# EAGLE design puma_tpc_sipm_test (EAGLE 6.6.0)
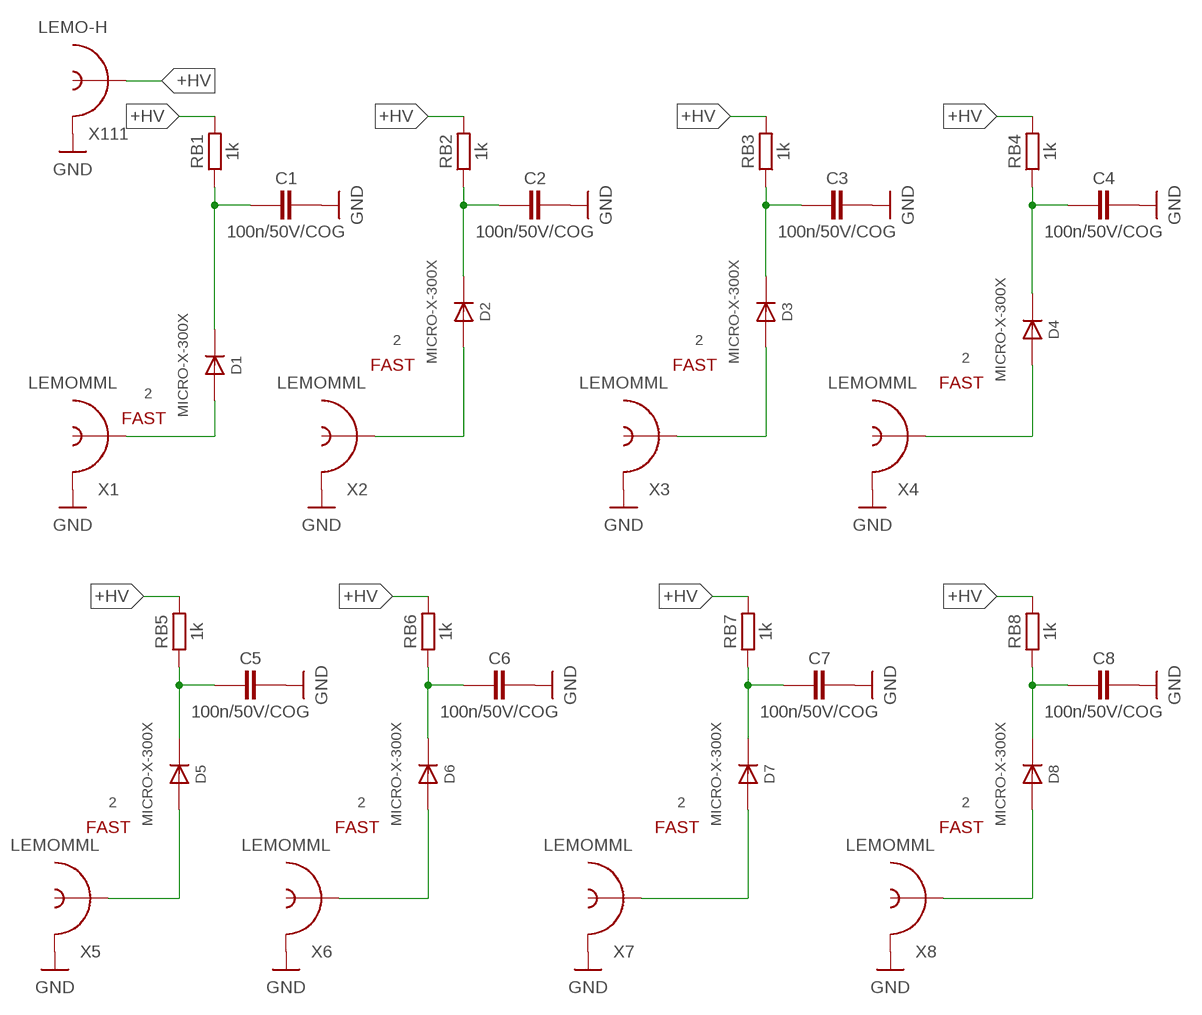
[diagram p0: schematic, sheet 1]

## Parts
C1  100n/50V/COG  C-EUCAP3216X130N  [CAP3216X130N]
C2  100n/50V/COG  C-EUCAP3216X130N  [CAP3216X130N]
C3  100n/50V/COG  C-EUCAP3216X130N  [CAP3216X130N]
C4  100n/50V/COG  C-EUCAP3216X130N  [CAP3216X130N]
C5  100n/50V/COG  C-EUCAP3216X130N  [CAP3216X130N]
C6  100n/50V/COG  C-EUCAP3216X130N  [CAP3216X130N]
C7  100n/50V/COG  C-EUCAP3216X130N  [CAP3216X130N]
C8  100n/50V/COG  C-EUCAP3216X130N  [CAP3216X130N]
D1  MICRO-X-300X  [MICROX-300XX]
D2  MICRO-X-300X  [MICROX-300XX]
D3  MICRO-X-300X  [MICROX-300XX]
D4  MICRO-X-300X  [MICROX-300XX]
D5  MICRO-X-300X  [MICROX-300XX]
D6  MICRO-X-300X  [MICROX-300XX]
D7  MICRO-X-300X  [MICROX-300XX]
D8  MICRO-X-300X  [MICROX-300XX]
RB1  1k  R-EU_RES1608X55N  [RES1608X55N]
RB2  1k  R-EU_RES1608X55N  [RES1608X55N]
RB3  1k  R-EU_RES1608X55N  [RES1608X55N]
RB4  1k  R-EU_RES1608X55N  [RES1608X55N]
RB5  1k  R-EU_RES1608X55N  [RES1608X55N]
RB6  1k  R-EU_RES1608X55N  [RES1608X55N]
RB7  1k  R-EU_RES1608X55N  [RES1608X55N]
RB8  1k  R-EU_RES1608X55N  [RES1608X55N]
X1  LEMOMML  [R302.302.000]
X2  LEMOMML  [R302.302.000]
X3  LEMOMML  [R302.302.000]
X4  LEMOMML  [R302.302.000]
X5  LEMOMML  [R302.302.000]
X6  LEMOMML  [R302.302.000]
X7  LEMOMML  [R302.302.000]
X8  LEMOMML  [R302.302.000]
X111  LEMO-H  [LEMO-H]

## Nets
+HV: RB1.2 RB2.2 RB3.2 RB4.2 RB5.2 RB6.2 RB7.2 RB8.2 X111.INNER
A1: D1.1(A) X1.1(INNER)
A2: D2.1(A) X2.1(INNER)
A3: D3.1(A) X3.1(INNER)
A4: D4.1(A) X4.1(INNER)
A5: D5.1(A) X5.1(INNER)
A6: D6.1(A) X6.1(INNER)
A7: D8.1(A) X8.1(INNER)
A8: D7.1(A) X7.1(INNER)
FILT1: C1.1 D1.3(K) RB1.1
FILT2: C2.1 D2.3(K) RB2.1
FILT3: C5.1 D5.3(K) RB5.1
FILT4: C6.1 D6.3(K) RB6.1
FILT9: C3.1 D3.3(K) RB3.1
FILT10: C4.1 D4.3(K) RB4.1
FILT11: C8.1 D8.3(K) RB8.1
FILT12: C7.1 D7.3(K) RB7.1
GND: C1.2 C2.2 C3.2 C4.2 C5.2 C6.2 C7.2 C8.2 X1.GND@1(SHIELD) X1.GND@2(SHIELD) X1.GND@3(SHIELD) X2.GND@1(SHIELD) X2.GND@2(SHIELD) X2.GND@3(SHIELD) X3.GND@1(SHIELD) X3.GND@2(SHIELD) X3.GND@3(SHIELD) X4.GND@1(SHIELD) X4.GND@2(SHIELD) X4.GND@3(SHIELD) X5.GND@1(SHIELD) X5.GND@2(SHIELD) X5.GND@3(SHIELD) X6.GND@1(SHIELD) X6.GND@2(SHIELD) X6.GND@3(SHIELD) X7.GND@1(SHIELD) X7.GND@2(SHIELD) X7.GND@3(SHIELD) X8.GND@1(SHIELD) X8.GND@2(SHIELD) X8.GND@3(SHIELD) X111.SHIELD@1(SHIELD) X111.SHIELD@2(SHIELD) X111.SHIELD@3(SHIELD) X111.SHIELD@4(SHIELD)
Unconnected: D1.2(FAST) D1.4(NC) D2.2(FAST) D2.4(NC) D3.2(FAST) D3.4(NC) D4.2(FAST) D4.4(NC) D5.2(FAST) D5.4(NC) D6.2(FAST) D6.4(NC) D7.2(FAST) D7.4(NC) D8.2(FAST) D8.4(NC)

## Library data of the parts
C1-C8 = rcl:C-EU: CAPACITOR, European symbol
D1-D8 = local:MICRO*-?: MPPC Diode with Fast output
RB1-RB8 = rcl:R-EU_: RESISTOR, European symbol
X1-X8 X111 = local:LEMO

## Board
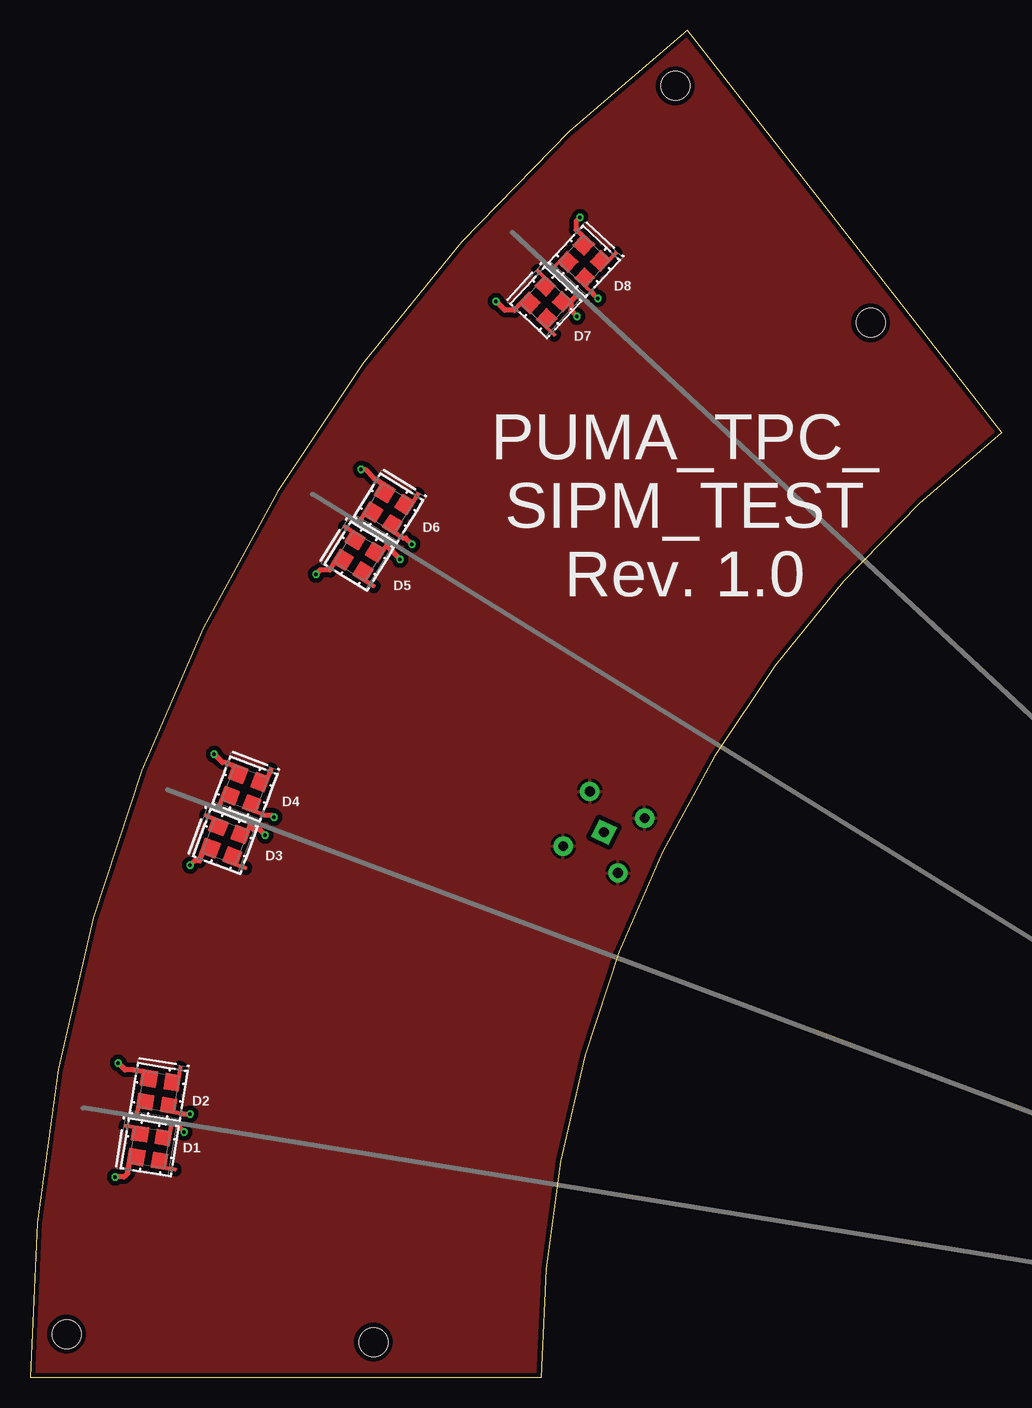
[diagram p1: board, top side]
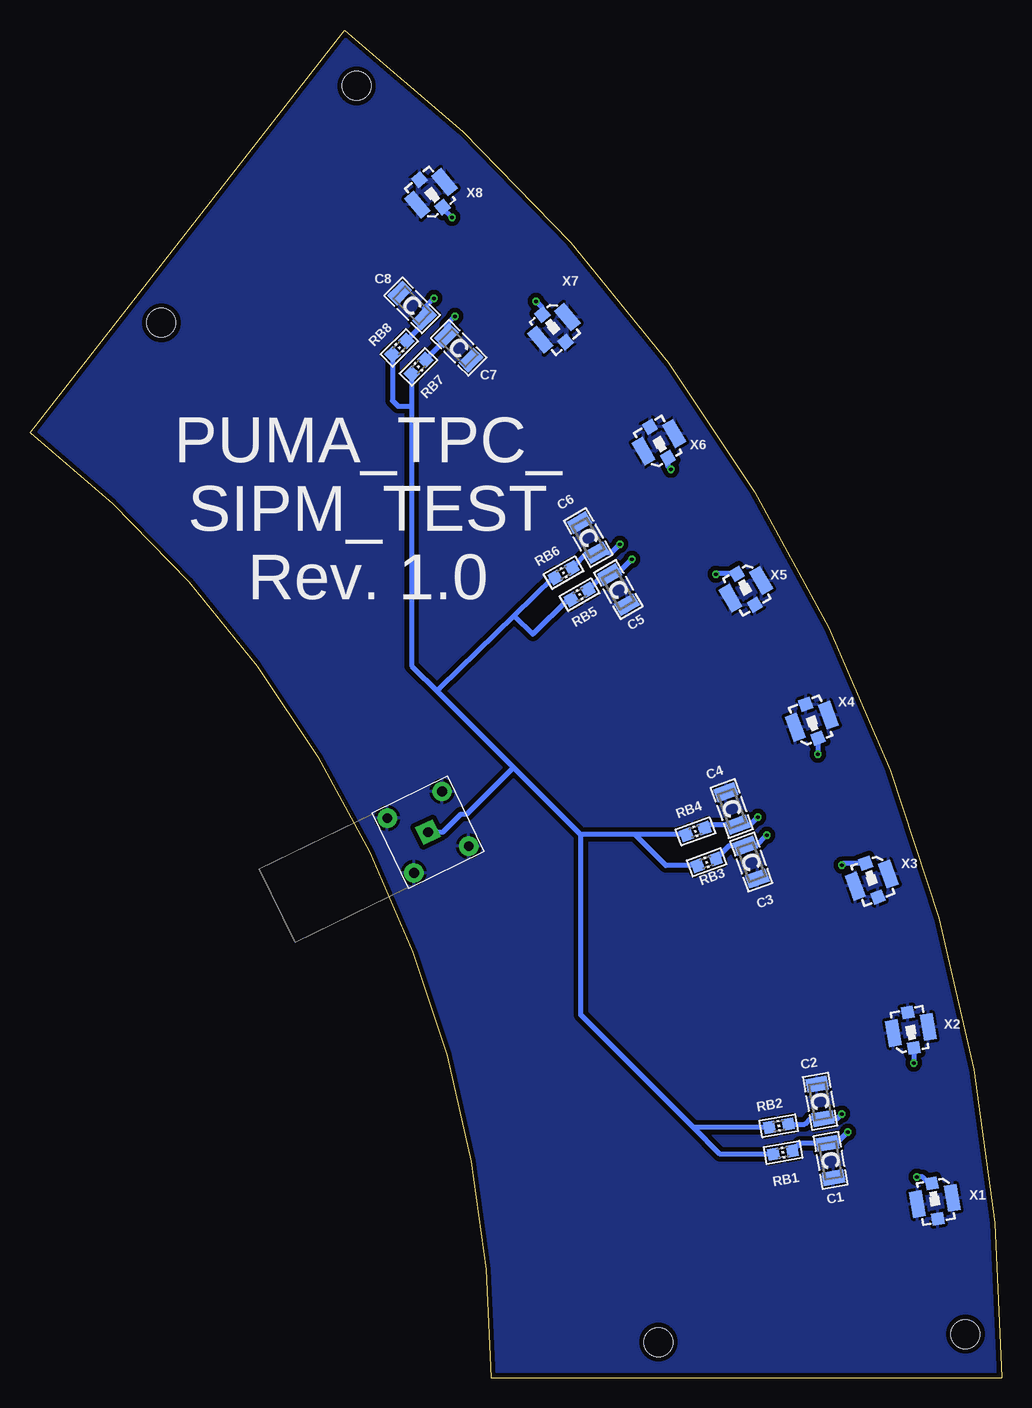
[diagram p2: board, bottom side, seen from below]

Size 81.03 x 112.37 mm. Coordinates in mm from the lower left corner, seen from the top.
Outline: 42.6,0 0,0 arc-52 54.81,112.37 81.03,78.8 arc52 42.6,0
Copper layers (1*16): Top 0.035mm / dielectric 1.5mm / Bottom 0.035mm
Design rules "l200_s150_d300_2l *": minimum track width 0.2mm, minimum drill 0.3mm, track to track 0.15mm, track to pad 0.15mm, pad to pad 0.15mm, via to via 0.15mm, smd to smd 0mil, copper to edge 0.4mm, drill to drill 0.5mm, minimum pad ring 0.4mm, minimum via ring 0.15mm, stop-mask expansion 0mil, vias tented up to drill 0mil, thermal gap 10mil
Holes 2.4 mm at 28.64,2.98 70.09,87.97 3.05,3.65 53.8,107.72

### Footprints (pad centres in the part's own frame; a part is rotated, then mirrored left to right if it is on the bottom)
CAP3216X130N = smd 1.15 x 1.8: 1 -1.45,0; 2 1.45,0
MICROX-300XX = smd 0.2 x 0.2: 1 -1.48,-2.28; 2 2.28,-1.48; 3 1.48,2.28; 4 -2.28,1.48
RES1608X55N = smd 0.95 x 1: 1 -0.8,0; 2 0.8,0
R302.302.000 = smd 1 x 1: 1 0,-1.5; GND@3 0,1.5 | smd 1.05 x 2.2: GND@1 1.475,0; GND@2 -1.475,0
LEMO-H = drill 0.813 pad 1.397 square: INNER 0,0 | drill 0.813 pad 1.397: SHIELD@1 -2.54,2.54; SHIELD@2 2.54,2.54; SHIELD@3 -2.54,-2.54; SHIELD@4 2.54,-2.54

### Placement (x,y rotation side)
C1  14.29,18.14 280 bottom
C2  15.16,23.06 100 bottom
C3  20.9,43.01 290 bottom
C4  22.52,47.47 110 bottom
C5  31.98,65.72 300 bottom
C6  34.48,70.05 120 bottom
C7  45.29,85.88 315 bottom
C8  49.18,89.41 135 bottom
D1  9.99,19.23 350.8 top
D2  10.74,23.84 260.8 top
D3  16.29,44.73 339.5 top
D4  17.92,49.11 249.3 top
D5  27.44,68.51 328.3 top
D6  29.9,72.49 238.3 top
D7  43.02,89.66 317 top
D8  46.21,93.08 227 top
RB1  18.25,18.8 190 bottom
RB2  18.6,21.02 190 bottom
RB3  24.61,42.98 200 bottom
RB4  25.55,45.57 200 bottom
RB5  35.21,65.3 210 bottom
RB6  36.55,67.12 210 bottom
RB7  48.65,84.29 225 bottom
RB8  50.24,85.88 225 bottom
X1  5.6,14.75 190 bottom
X2  7.6,29 10 bottom
X3  10.85,41.5 200 bottom
X4  15.85,54.75 20 bottom
X5  21.35,65.75 210 bottom
X6  28.6,78 30 bottom
X7  37.35,87.5 220 bottom
X8  47.6,98.75 40 bottom
X111  47.85,45.5 206 bottom

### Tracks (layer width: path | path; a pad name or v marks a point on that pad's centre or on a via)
+HV
  Bottom 0.4: RB7.2 49.21,81 | 49.21,81 49.21,59.36 46.97,57.12 | 46.97,57.12 40.72,50.88 | 40.72,50.88 35.14,45.29 | RB4.2 30.6,45.29 | 30.6,45.29 35.14,45.29 | RB6.2 37.38,66.72 40.62,63.56 | 40.62,63.56 46.85,57.5 46.97,57.38 46.97,57.12 | RB2.2 25.73,20.88 | 25.73,20.88 35.1,30.25 35.1,45.25 35.14,45.29 | RB3.2 28.02,42.71 30.6,45.29 | RB1.2 23.51,18.66 25.73,20.88 | RB5.2 36.2,64.9 39.1,62 40.62,63.52 40.62,63.56 | RB8.2 50.8,81.45 50.35,81 49.21,81 | X111.INNER 46.6,45.5 45.1,47 44.6,47 40.72,50.88
A1  (via drill 0.3)
  Top 0.4: D1.1 8.16,17.06 7.85,16.75 v7.1,16.75
  Bottom 0.4: X1.1 6.08,16.23 6.6,16.75 v7.1,16.75
A2  (via drill 0.3)
  Top 0.4: D2.1 7.93,25.67 v7.35,26.25
  Bottom 0.4: X2.1 v7.34,26.26 v7.35,26.25
A3  (via drill 0.3)
  Top 0.4: D3.1 13.71,43.11 v13.35,42.75
  Bottom 0.4: X3.1 13.19,42.91 v13.35,42.75
A4  (via drill 0.3)
  Top 0.4: D4.1 16.05,51.3 v15.35,52
  Bottom 0.4: X4.1 15.34,52.01 v15.35,52
A5  (via drill 0.3)
  Top 0.4: D5.1 24.2,67.35 v23.85,67
  Bottom 0.4: X5.1 23.8,67.05 v23.85,67
A6  (via drill 0.3)
  Top 0.4: v27.6,75.75 27.94,75.75 D6.1
  Bottom 0.4: X6.1 27.85,76 v27.6,75.75
A7  (via drill 0.3)
  Top 0.4: D8.1 45.55,96.45 v45.85,96.75
  Bottom 0.4: X8.1 46.64,97.54 v45.85,96.75
A8  (via drill 0.3)
  Top 0.4: D7.1 39.59,89 v38.85,89.75
  Bottom 0.4: X7.1 38.31,89.21 v38.85,89.75
FILT1  (via drill 0.3)
  Top 0.4: D1.3 12.11,21.24 v12.85,20.5
  Bottom 0.4: v12.85,20.5 13.79,19.56 C1.1 16.84,19.56 RB1.1
FILT2  (via drill 0.3)
  Top 0.4: D2.3 13.33,22.02 v13.35,22
  Bottom 0.4: v13.35,22 13.72,21.63 C2.1 15.97,21.63 16.44,21.16 RB2.1
FILT3  (via drill 0.3)
  Top 0.4: D5.3 29.9,69.3 29.85,69.25 v30.85,68.25
  Bottom 0.4: v30.85,68.25 32.12,66.97 C5.1 33.24,66.97 RB5.1
FILT4  (via drill 0.3)
  Top 0.4: D6.3 31.32,70.03 v31.85,69.5
  Bottom 0.4: v31.85,69.5 32.56,68.79 C6.1 34.59,68.79 RB6.1
FILT9  (via drill 0.3)
  Top 0.4: D3.3 18.47,45.88 18.6,45.75 19.1,45.75 v19.6,45.25
  Bottom 0.4: v19.6,45.25 20.48,44.37 C3.1 22.75,44.37 RB3.1
FILT10  (via drill 0.3)
  Top 0.4: D4.3 20.18,46.92 v20.35,46.75
  Bottom 0.4: v20.35,46.75 20.99,46.11 C4.1 24.74,46.11 25.1,45.75 24.89,45.75 RB4.1
FILT11  (via drill 0.3)
  Top 0.4: D8.3 46.9,90.45 v47.35,90
  Bottom 0.4: v47.35,90 48.15,89.2 C8.1 48.15,87.97 RB8.1
FILT12  (via drill 0.3)
  Top 0.4: D7.3 45.66,90.31 45.1,89.75 45.1,89 v45.6,88.5
  Bottom 0.4: v45.6,88.5 46.31,87.78 C7.1 46.31,86.62 RB7.1
GND
  pour Bottom (isolate 0.4): -1.4,-1 82.6,-1 82.6,115 -1.4,115
  pour Top (isolate 0.4): -1.4,-1 82.6,-1 82.6,115 -1.4,115

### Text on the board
tPlace: PUMA_TPC_ / SIPM_TEST / Rev. 1.0
bPlace: PUMA_TPC_ / SIPM_TEST / Rev. 1.0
